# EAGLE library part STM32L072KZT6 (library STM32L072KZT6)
ARM Microcontrollers - MCU Ultra-low-power ARM Cortex-M0+ MCU with 192-Kbytes Flash, 32 MHz CPU, USB Source: Datasheet
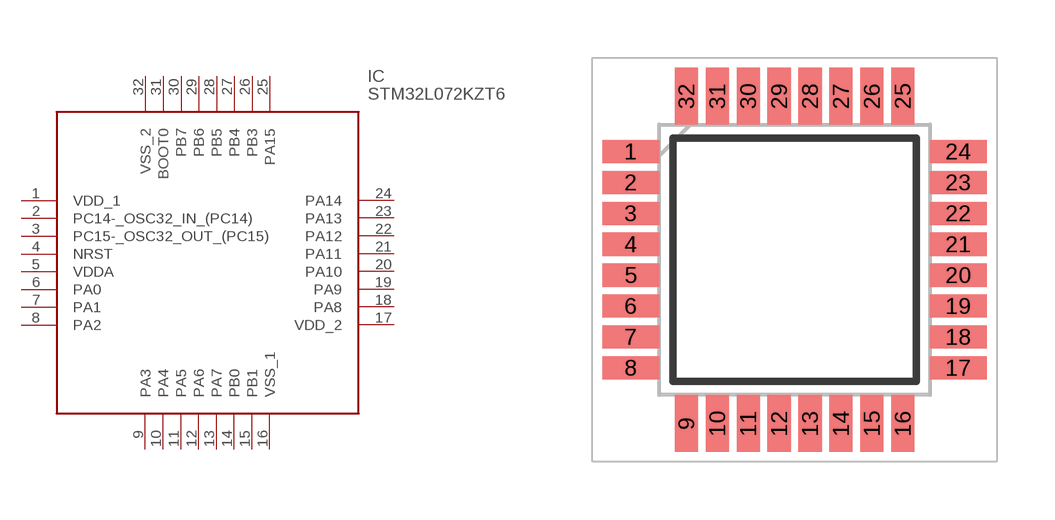
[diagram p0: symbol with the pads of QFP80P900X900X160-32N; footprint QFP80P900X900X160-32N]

Designator prefix IC

## STM32L072KZT6 (Description: ARM Microcontrollers - MCU Ultra-low-power ARM Cortex-M0+ MCU with 192-Kbytes Flash, 32 MHz CPU, USB; Height: 1.6mm; Manufacturer_Name: STMicroelectronics; Manufacturer_Part_Number: STM32L072KZT6; Mouser_Part_Number: 511-STM32L072KZT6; Mouser_Price-Stock: https://www.mouser.co.uk/ProductDetail/STMicroelectronics/STM32L072KZT6?qs=mwoc%252BQmZlGJ4eN3sEity4A%3D%3D)  [QFP80P900X900X160-32N]
1  VDD_1
2  PC14-_OSC32_IN_(PC14)
3  PC15-_OSC32_OUT_(PC15)
4  NRST
5  VDDA
6  PA0
7  PA1
8  PA2
9  PA3
10  PA4
11  PA5
12  PA6
13  PA7
14  PB0
15  PB1
16  VSS_1
17  VDD_2
18  PA8
19  PA9
20  PA10
21  PA11
22  PA12
23  PA13
24  PA14
25  PA15
26  PB3
27  PB4
28  PB5
29  PB6
30  PB7
31  BOOT0
32  VSS_2

## Footprint QFP80P900X900X160-32N (pad centres in mm)
ST LQFP32
smd 1.475 x 0.6: 1 -4.238,2.8; 2 -4.238,2; 3 -4.238,1.2; 4 -4.238,0.4; 5 -4.238,-0.4; 6 -4.238,-1.2; 7 -4.238,-2; 8 -4.238,-2.8; 17 4.238,-2.8; 18 4.238,-2; 19 4.238,-1.2; 20 4.238,-0.4; 21 4.238,0.4; 22 4.238,1.2; 23 4.238,2; 24 4.238,2.8
smd 0.6 x 1.475: 9 -2.8,-4.238; 10 -2,-4.238; 11 -1.2,-4.238; 12 -0.4,-4.238; 13 0.4,-4.238; 14 1.2,-4.238; 15 2,-4.238; 16 2.8,-4.238; 25 2.8,4.238; 26 2,4.238; 27 1.2,4.238; 28 0.4,4.238; 29 -0.4,4.238; 30 -1.2,4.238; 31 -2,4.238; 32 -2.8,4.238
